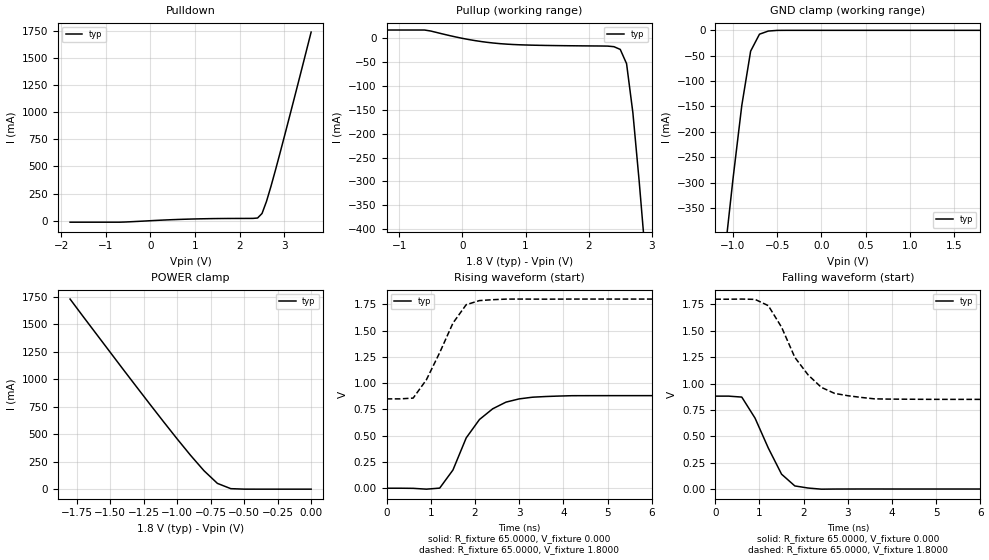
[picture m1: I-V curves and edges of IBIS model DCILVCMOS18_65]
| / 7\'7
| \ \   Xilinx Inc.
| / /
| \_\/.\   IBIS Model for Virtex-II
[IBIS ver]   2.1
[File name]   dci1865.ibs
[File Rev]   1.1
[Date]   Aug. 1, 2001
[Source]   Hspice simulations (08-1: TT, SS, FF)
[Notes]   Xilinx IBIS model for LVDCI 1.8V 65 ohms driver
[Disclaimer] The data in this model is derived from SPICE simulations using
   modeling information extracted from the target process. While
   a great deal of care has been taken to provide information
   that is accurate, this model is considered preliminary as it
   has not been verified by actual silicon measurement. Treat the
   data in this model as preliminary until actual silicon
   verification is performed.
[Copyright]   Copyright 2001, Xilinx Inc., All rights reserved
|   Component Virtex_II
[Component]   Virtex_II
[Manufacturer]   Xilinx Inc.
[Package]
| variable   typ   min   max
R_pkg   0.1000   NA   NA
L_pkg   0.8000nH   NA   NA
C_pkg   0.5000pF   NA   NA
[Pin]  signal_name   model_name   R_pin   L_pin   C_pin
io   DCILVCMOS18_65   DCILVCMOS18_65
| ins  insig   inp
| ens  ensig   inp
PGND   GND   GND
VCCO   VCCO   POWER
| Models and submodels in the file (1): DCILVCMOS18_65 (I/O)
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|   Model DCILVCMOS18_65
[Model]   DCILVCMOS18_65
Model_type   I/O
Polarity   Non-Inverting
Enable   Active-Low
Vinh = 1.19V
Vinl = 0.4V
Vmeas =   0.7900V
Cref =  35.0000pF
Rref =   1.0000M
Vref =  0.000V
C_comp   7.0000pF   NA   NA
[Temperature Range]   25.0000   NA   NA
[Voltage Range]   1.8000V   NA   NA
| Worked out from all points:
|   slope of the pulldown table from 0 to 0.27 V, typ, clamps not added: 47.8 ohm
|   slope of the pullup table from 0 to 0.27 V, typ, clamps not added: 44 ohm
|   GND clamp passes 1 mA (typ) near -0.57 V on its own axis
|   POWER clamp passes 1 mA (typ) near -0.52 V on its own axis
|   rising waveform, R_fixture 65.0000, V_fixture 0.000: 20-80 % time 747ps typ, NA min, NA max; typ from 0 V to 0.881 V
|   rising waveform, R_fixture 65.0000, V_fixture 1.8000: 20-80 % time 657ps typ, NA min, NA max; typ from 0.85 V to 1.8 V
|   falling waveform, R_fixture 65.0000, V_fixture 0.000: 20-80 % time 606ps typ, NA min, NA max; typ from 0.881 V to 0 V
|   falling waveform, R_fixture 65.0000, V_fixture 1.8000: 20-80 % time 818ps typ, NA min, NA max; typ from 1.8 V to 0.85 V
[Pulldown]
| voltage   I(typ)   I(min)   I(max)
-1.8V     -13.61mA   NA         NA
-700mV    -13.61mA   NA         NA
800mV     14.01mA    NA         NA
2.4V      24.86mA    NA         NA
2.5V      66.76mA    NA         NA
2.6V      178mA      NA         NA
2.7V      316.7mA    NA         NA
3V        775.5mA    NA         NA
3.6V      1.738A     NA         NA
[Pullup]
| voltage   I(typ)   I(min)   I(max)
-1.8V     17.46mA    NA         NA
-600mV    17.46mA    NA         NA
100mV     -2.499mA   NA         NA
500mV     -9.941mA   NA         NA
2.3V      -16.24mA   NA         NA
2.4V      -17.46mA   NA         NA
2.5V      -23.2mA    NA         NA
2.6V      -53.01mA   NA         NA
2.7V      -155.8mA   NA         NA
2.8V      -299.8mA   NA         NA
2.9V      -457.9mA   NA         NA
3.6V      -1.654A    NA         NA
[GND_clamp]
| voltage   I(typ)   I(min)   I(max)
-1.8V     -1.649A    NA         NA
-1.1V     -452.1mA   NA         NA
-1V       -293.4mA   NA         NA
-900mV    -148mA     NA         NA
-800mV    -41.01mA   NA         NA
-700mV    -7.602mA   NA         NA
-600mV    -1.419mA   NA         NA
-500mV    -128.9uA   NA         NA
1.8V      272.1nA    NA         NA
[POWER_clamp]
| voltage   I(typ)   I(min)   I(max)
-1.8V     1.731A     NA         NA
-1.4V     1.085A     NA         NA
-1V       456.9mA    NA         NA
-800mV    167.8mA    NA         NA
-700mV    52.78mA    NA         NA
-600mV    4.607mA    NA         NA
0V        272.1nA    NA         NA
[Ramp]
| variable   typ   min   max
dV/dt_r   0.5285/0.7909n   NA   NA
dV/dt_f   0.5699/0.8767n   NA   NA
R_load = 65.0000
[Rising Waveform]
R_fixture = 65.0000
V_fixture = 0.000
| time   V(typ)   V(min)   V(max)
0s        10.53uV    NA         NA
1.2ns     889.7uV    NA         NA
1.5ns     173.2mV    NA         NA
1.8ns     478.8mV    NA         NA
2.1ns     653.8mV    NA         NA
2.4ns     755.9mV    NA         NA
2.7ns     819.2mV    NA         NA
3ns       850.1mV    NA         NA
4.2ns     880.4mV    NA         NA
15ns      880.9mV    NA         NA
[Rising Waveform]
R_fixture = 65.0000
V_fixture = 1.8000
V_fixture_min = 1.7000
V_fixture_max = 1.9000
| time   V(typ)   V(min)   V(max)
0s        850.1mV    NA         NA
600ps     857.7mV    NA         NA
900ps     1.032V     NA         NA
1.2ns     1.29V      NA         NA
1.5ns     1.571V     NA         NA
1.8ns     1.746V     NA         NA
2.1ns     1.786V     NA         NA
2.7ns     1.8V       NA         NA
3ns       1.8V       NA         NA
15ns      1.8V       NA         NA
[Falling Waveform]
R_fixture = 65.0000
V_fixture = 0.000
| time   V(typ)   V(min)   V(max)
0s        880.9mV    NA         NA
300ps     880.9mV    NA         NA
600ps     871.8mV    NA         NA
900ps     672.2mV    NA         NA
1.2ns     388.4mV    NA         NA
1.5ns     140.5mV    NA         NA
1.8ns     29.17mV    NA         NA
2.1ns     9.371mV    NA         NA
2.4ns     -1.481mV   NA         NA
15ns      -7.201uV   NA         NA
[Falling Waveform]
R_fixture = 65.0000
V_fixture = 1.8000
V_fixture_min = 1.7000
V_fixture_max = 1.9000
| time   V(typ)   V(min)   V(max)
0s        1.8V       NA         NA
900ps     1.798V     NA         NA
1.2ns     1.739V     NA         NA
1.5ns     1.535V     NA         NA
1.8ns     1.248V     NA         NA
2.1ns     1.083V     NA         NA
2.4ns     964mV      NA         NA
3ns       884.7mV    NA         NA
3.9ns     852.8mV    NA         NA
15ns      850.1mV    NA         NA
